ORGANIZATION_BLOCK OB 1
	TITLE		= This is the title
	{ attribute1 := 'value 1';
	  attribute2 := 'value 2' }
	AUTHOR		: This is the author
	FAMILY		: This is the family
	NAME		: This is the name
	VERSION		: 0.1
	VAR_TEMP
		// Temporary variables
	END_VAR
BEGIN
NETWORK
	TITLE = This is the first network title
	NOP 0
NETWORK
	TITLE = This is the second network title
	NOP 0


	CALL SFC 46 // STOP CPU
END_ORGANIZATION_BLOCK


FUNCTION FC 1: VOID
	TITLE		= This is the title
	{ attribute1 := 'value 1';  attribute2 := 'value 2' }
	AUTHOR		: This is the author
	FAMILY		: This is the family
	NAME		: This is the name
	VERSION		: 0.1
	VAR_INPUT
		// Input variables
	END_VAR
	VAR_OUTPUT
		// Output variables
	END_VAR
	VAR_IN_OUT
		// Input/output variables
	END_VAR
	VAR_TEMP
		// Temporary variables
	END_VAR
BEGIN
NETWORK
	TITLE = This is the first network title
	NOP 0
NETWORK
	TITLE = This is the second network title
	NOP 0
END_FUNCTION


FUNCTION_BLOCK FB 1
	TITLE		= This is the title
	{ attribute1 := 'value 1';  attribute2 := 'value 2' }
	AUTHOR		: This is the author
	FAMILY		: This is the family
	NAME		: This is the name
	VERSION		: 0.1
	VAR
		// Static variables
	END_VAR
	VAR_INPUT
		// Input variables
	END_VAR
	VAR_OUTPUT
		// Output variables
	END_VAR
	VAR_IN_OUT
		// Input/output variables
	END_VAR
	VAR_TEMP
		// Temporary variables
	END_VAR
BEGIN
NETWORK
	TITLE = This is the first network title
	NOP 0
NETWORK
	TITLE = This is the second network title
	NOP 0
END_FUNCTION_BLOCK


DATA_BLOCK DB 1
	TITLE		= This is the title
	AUTHOR		: This is the author
	FAMILY		: This is the family
	NAME		: This is the name
	VERSION		: 0.1
	STRUCT
		// Data structure
	END_STRUCT
BEGIN
END_DATA_BLOCK


DATA_BLOCK DB 2
	FB 1
	TITLE		= This is the title
	AUTHOR		: This is the author
	FAMILY		: This is the family
	NAME		: This is the name
	VERSION		: 0.1
BEGIN
END_DATA_BLOCK


DATA_BLOCK DB 3
	SFB -1
	TITLE		= This is the title
	AUTHOR		: This is the author
	FAMILY		: This is the family
	NAME		: This is the name
	VERSION		: 0.1
BEGIN
END_DATA_BLOCK
